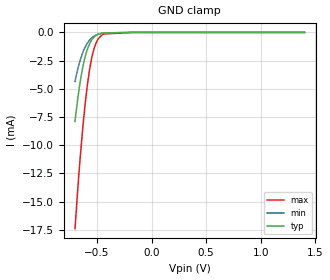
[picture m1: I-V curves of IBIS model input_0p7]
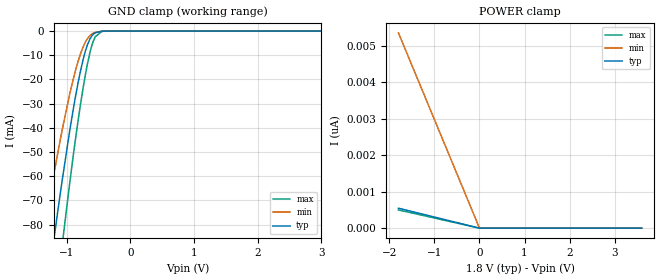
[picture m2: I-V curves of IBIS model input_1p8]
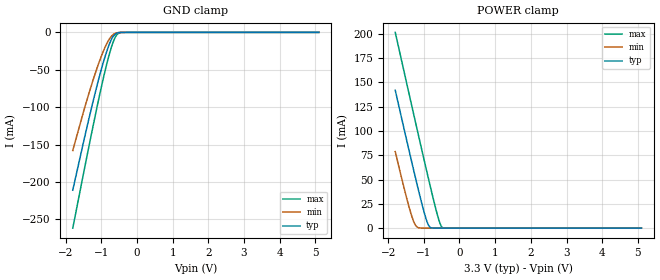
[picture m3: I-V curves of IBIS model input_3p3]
|Texas Instruments Incorporated
|1-Bit Dual-Supply Bus Transceiver With Configurable Voltage Translation
|and 3-State Outputs
| Marketing part#   Digital Voltage Range   Package-type   #pins
| SN74AXC1T45DBV   0.65V-3.6V   SOT   6
| SN74AXC1T45DRL   0.65V-3.6V   SOT   6
| SN74AXC1T45DCK   0.65V-3.6V   SOT   6
| SN74AXC1T45DSF   0.65V-3.6V   X2SON   6
| SN74AXC1T45DTB   0.65V-3.6V   X2SON   6
[IBIS Ver]   4.1
[File name]   sn74axc1t45.ibs
[Date]   02/22/2019
[File Rev]   1.1
[Source]
| Texas Instruments Incorporated.
| Analog-eLab Design Center, HPA
| 12500 TI Blvd
| Dallas, TX -75243
[Notes]
| Rev 1.1: 02/22/2019
| - Added input_1p8 and io_1p8 model.
| Rev 1.0: 10/26/2017
| - Initial version of the model
| - Model generated from simulations in SPECTRE
| - Model matched to SPICE simulation
| - C_comp although listed in numerical order of value are
|   obtained from varying PVT conditions. For PVT conditions for
|   each specific value refer the buffer description under
|   respective [Model]. IBIS model user is responsible for using
|   appropriate C_comp to simulate for Signal Integrity.
[Disclaimer]
| This model is designed as an aid for customers of Texas Instruments.
| TI and its licensors and suppliers make no warranties, either expressed
| or implied, with respect to this  model, including the warranties of
| merchantability or fitness for a particular purpose. The model is
| provided solely on an "as is" basis. The entire risk as to its quality
| and performance is with the customer.
[Copyright]
(C) Copyright 2019 Texas Instruments Incorporated.All rights reserved.
|Component SN74AXC1T45DBV 6-pin SOT - DBV package
|  Part # SN74AXC1T45DBV
[Component]   SN74AXC1T45DBV
[Manufacturer]  TI
[Package]   |6 SOT - DBV package
|   typ   min   max
R_pkg   0.05   0.04   0.06
L_pkg   1.0nH   0.8nH   1.2nH
C_pkg   0.2pF   0.16pF   0.24pF
[Pin]  signal_name model_name   R_pin   L_pin   C_pin
1   VCCA   power   NA   NA   NA
2   GND   gnd   NA   NA   NA
3   A   io   NA   NA   NA
4   B   io   NA   NA   NA
5   DIR   input   NA   NA   NA
6   VCCB   power   NA   NA   NA
|Component SN74AXC1T45DRL 6-pin SOT - DRL package
|  Part # SN74AXC1T45DRL
[Component]   SN74AXC1T45DRL
[Manufacturer]  TI
[Package]   |6 SOT - DRL package
|   typ   min   max
R_pkg   0.05   0.04   0.06
L_pkg   1.0nH   0.8nH   1.2nH
C_pkg   0.2pF   0.16pF   0.24pF
[Pin]  signal_name model_name   R_pin   L_pin   C_pin
1   VCCA   power   NA   NA   NA
2   GND   gnd   NA   NA   NA
3   A   io   NA   NA   NA
4   B   io   NA   NA   NA
5   DIR   input   NA   NA   NA
6   VCCB   power   NA   NA   NA
|Component SN74AXC1T45DCK 6-pin SOT - DCK package
|  Part # SN74AXC1T45DCK
[Component]   SN74AXC1T45DCK
[Manufacturer]  TI
[Package]   |6 SOT - DCK package
|   typ   min   max
R_pkg   0.05   0.04   0.06
L_pkg   1.0nH   0.8nH   1.2nH
C_pkg   0.2pF   0.16pF   0.24pF
[Pin]  signal_name model_name   R_pin   L_pin   C_pin
1   VCCA   power   NA   NA   NA
2   GND   gnd   NA   NA   NA
3   A   io   NA   NA   NA
4   B   io   NA   NA   NA
5   DIR   input   NA   NA   NA
6   VCCB   power   NA   NA   NA
|Component SN74AXC1T45DSF 6-pin SOT - DSF package
|  Part # SN74AXC1T45DSF
[Component]   SN74AXC1T45DSF
[Manufacturer]  TI
[Package]   |6 X2SON - DSF package
|   typ   min   max
R_pkg   0.05   0.04   0.06
L_pkg   1.0nH   0.8nH   1.2nH
C_pkg   0.2pF   0.16pF   0.24pF
[Pin]  signal_name model_name   R_pin   L_pin   C_pin
1   VCCA   power   NA   NA   NA
2   GND   gnd   NA   NA   NA
3   A   io   NA   NA   NA
4   B   io   NA   NA   NA
5   DIR   input   NA   NA   NA
6   VCCB   power   NA   NA   NA
|Component SN74AXC1T45DTB 6-pin SOT - DTB package
|  Part # SN74AXC1T45DTB
[Component]   SN74AXC1T45DTB
[Manufacturer]  TI
[Package]   |6 X2SON -  DTB package
|   typ   min   max
R_pkg   0.05   0.04   0.06
L_pkg   1.0nH   0.8nH   1.2nH
C_pkg   0.2pF   0.16pF   0.24pF
[Pin]  signal_name model_name   R_pin   L_pin   C_pin
1   VCCA   power   NA   NA   NA
2   GND   gnd   NA   NA   NA
3   A   io   NA   NA   NA
4   B   io   NA   NA   NA
5   DIR   input   NA   NA   NA
6   VCCB   power   NA   NA   NA
|   Model Selectors
[Model Selector] input
input_0p7   0.7V   digital Input
input_1p8   1.8V   digital Input
input_3p3   3.3V   digital Input
[Model Selector] io
io_0p7   0.7V   digital I/O
io_1p8   1.8V   digital I/O
io_3p3   3.3V   digital I/O
| Models and submodels in the file (6): input_0p7 (Input), input_1p8 (Input), input_3p3 (Input), io_0p7 (I/O), io_1p8 (I/O), io_3p3 (I/O)
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|   input_0p7 Model
[Model]   input_0p7
Model_type   Input
Vinl = 0.21
Vinh = 0.49
|   typ   min   max
C_comp   7.40696E-13   6.45127E-13   8.98734E-13
[Model spec]
|subparameter
Vinl   0.21   0.195   0.225
Vinh   0.49   0.455   0.525
| Where Nom  PVT is Nominal Process, 0.7V, 27C
|   Fast PVT is Strong Process,  0.75V, -40C
|   Slow PVT is Weak Process,   0.65, 130C
[Voltage Range]   0.7   0.65   0.75
|Junction Temperature
[Temperature Range]   27   130   -40
[Power Clamp Reference]   0.7   0.65   0.75
[GND Clamp Reference]   0   0   0
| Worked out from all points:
|   GND clamp passes 1 mA (typ) near -0.57 V on its own axis
[GND Clamp]
|   Voltage   I(typ)   I(min)   I(max)
-700mV    -7.896mA   -4.354mA   -17.4mA
-676.9mV  -6.033mA   -3.335mA   -14.2mA
-651.7mV  -4.329mA   -2.43mA    -11.02mA
-624.4mV  -2.873mA   -1.673mA   -7.992mA
-588.7mV  -1.545mA   -978.4uA   -4.797mA
-567.7mV  -1.026mA   -696.2uA   -3.358mA
-548.8mV  -691.6uA   -504.6uA   -2.342mA
-527.8mV  -434.7uA   -346.8uA   -1.503mA
-487.9mV  -168.3uA   -161.7uA   -574.9uA
-454.3mV  -71.1uA    -80.61uA   -230.7uA
-175mV    -4.456nA   -77.57nA   0A
1.4V      0A         0A         0A
[POWER Clamp]
|   Voltage   I(typ)   I(min)   I(max)
-700mV    0A         0A         0A
0V        0A         0A         0A
1.4V      0A         0A         0A
|   input_1p8 Model
[Model]   input_1p8
Model_type   Input
Vinl = 0.7
Vinh = 1.6
|   typ   min   max
C_comp   1.392pf   0.843pf   1.994pF
| Where Nom  PVT is Nominal Process, 1.8V,  27C
|   Fast PVT is Strong Process,  1.98V, -40C
|   Slow PVT is Weak Process,   1.62V, 130C
[Voltage Range]   1.8   1.62   1.98
|Junction Temperature
[Temperature Range]   27   130   -40
[Power Clamp Reference]   1.8   1.62   1.98
[GND Clamp Reference]   0   0   0
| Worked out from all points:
|   GND clamp passes 1 mA (typ) near -0.56 V on its own axis
[GND Clamp]
|   Voltage   I(typ)   I(min)   I(max)
-1.8V     -210.9mA   -157.9mA   -261.6mA
-1.319V   -109.8mA   -77.26mA   -146mA
-1.206V   -87.46mA   -60.12mA   -119.6mA
-1.12V    -71.04mA   -47.78mA   -99.81mA
-1.066V   -61.14mA   -40.45mA   -87.72mA
-952.2mV  -41.52mA   -26.26mA   -63.25mA
-903.6mV  -33.72mA   -20.8mA    -53.27mA
-779.4mV  -16.26mA   -9.28mA    -30.01mA
-676.8mV  -6.025mA   -3.331mA   -14.19mA
-579.6mV  -1.299mA   -846.1uA   -4.132mA
-385.2mV  -10.15uA   -16.94uA   -26.09uA
3.6V      0A         0A         0A
[POWER Clamp]
|   Voltage   I(typ)   I(min)   I(max)
-1.8V     546.7pA    5.348nA    499.5pA
0V        0A         0A         0A
3.6V      0A         0A         0A
|   input_3p3 Model
[Model]   input_3p3
Model_type   Input
Vinl = 0.8
Vinh = 2.3
|   typ   min   max
C_comp   1.86062E-12   1.26954E-12   2.13619E-12
| Where Nom  PVT is Nominal Process, 3.3V, 27C
|   Fast PVT is Strong Process,  3.6V, -40C
|   Slow PVT is Weak Process,   3.0V, 130C
[Voltage Range]   3.3   3   3.6
|Junction Temperature
[Temperature Range]   27   130   -40
[Power Clamp Reference]   3.3   3   3.6
[GND Clamp Reference]   0   0   0
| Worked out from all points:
|   GND clamp passes 1 mA (typ) near -0.57 V on its own axis
|   POWER clamp passes 1 mA (typ) near -0.83 V on its own axis
[GND Clamp]
|   Voltage   I(typ)   I(min)   I(max)
-1.8V     -210.9mA   -157.9mA   -261.6mA
-1.49V    -144.7mA   -104.6mA   -186.5mA
-1.296V   -105.2mA   -73.69mA   -140.6mA
-1.117V   -70.54mA   -47.4mA    -99.2mA
-951.3mV  -41.37mA   -26.15mA   -63.06mA
-820.2mV  -21.52mA   -12.61mA   -37.23mA
-716.7mV  -9.415mA   -5.207mA   -19.86mA
-613.2mV  -2.39mA    -1.422mA   -6.892mA
-523.5mV  -394uA     -320.5uA   -1.365mA
-426.9mV  -33.77uA   -44.18uA   -102.3uA
-68.1mV   0A         0A         0A
5.1V      0A         0A         0A
[POWER Clamp]
|   Voltage   I(typ)   I(min)   I(max)
-1.8V     141.9mA    78.74mA    201.4mA
-1.414V   79.93mA    21.78mA    138.3mA
-1.296V   61.5mA     8.016mA    119.2mA
-1.234V   51.89mA    3.123mA    109.2mA
-1.151V   39.29mA    456.6uA    95.81mA
-985.8mV  15.65mA    4.189uA    69.3mA
-868.5mV  3.093mA    131.9nA    50.79mA
-799.5mV  400.9uA    7.757nA    40.08mA
-571.8mV  47.54nA    0A         7.669mA
-516.6mV  0A         0A         2.383mA
-468.3mV  0A         0A         390.4uA
5.1V      0A         0A         0A
